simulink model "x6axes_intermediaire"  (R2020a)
settings: Solver=FixedStepAuto  StartTime=0.0  StopTime=t(numel(t))  FixedStep=dt  RelTol=1e-3
model workspace: external: MATLAB File (data not in the file)
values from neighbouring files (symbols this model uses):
  X = [X1(:,1:numel(X1(1,:))-1) X2]    [concat_motion.m]    (also in MGD_6axes.m = [T(1:3,4);Euler]; Trace_6axes.m = [0 0 0; Trace_6axes_trajectoire.m = [0 0 0)
undefined symbols (not defined in the file or in its folder): deg, kg, m, mm, N, rad, s, smiData, Y, Z
libraries: sm_lib x37, nesl_utility x10

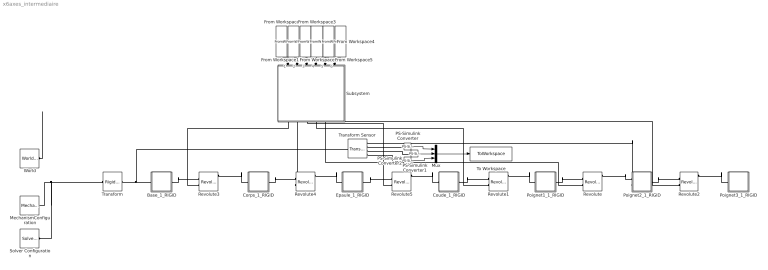
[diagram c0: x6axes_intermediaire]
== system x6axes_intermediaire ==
  Base_1_RIGID : Subsystem
  Corps_1_RIGID : Subsystem
  Coude_1_RIGID : Subsystem
  Epaule_1_RIGID : Subsystem
  From Workspace : FromWorkspace  VariableName=[t' q_targ(1,:)']
  From Workspace1 : FromWorkspace  VariableName=[t' q_targ(2,:)']
  From Workspace2 : FromWorkspace  VariableName=[t' q_targ(3,:)']
  From Workspace3 : FromWorkspace  VariableName=[t' q_targ(4,:)']
  From Workspace4 : FromWorkspace  VariableName=[t' q_targ(5,:)']
  From Workspace5 : FromWorkspace  VariableName=[t' q_targ(6,:)']
  MechanismConfiguration : sm_lib/Utilities/Mechanism Configuration  UniformGravity=Constant  GravityVector=[0 0 -9.80665]  GravityUnits=m/s^2  LinearizationDelta=0.001
  Mux : Mux  Inputs=3
  PS-Simulink Converter : nesl_utility/PS-Simulink Converter  PhysicalDomain=network_engine_domain  SubClassName=ps_output  LeftPortType=input  RightPortType=output  PseudoPeriodic=off  Frequencies=[]  Unit=m  AffineConversion=off
  PS-Simulink Converter1 : nesl_utility/PS-Simulink Converter  PhysicalDomain=network_engine_domain  SubClassName=ps_output  LeftPortType=input  RightPortType=output  PseudoPeriodic=off  Frequencies=[]  Unit=m  AffineConversion=off
  PS-Simulink Converter2 : nesl_utility/PS-Simulink Converter  PhysicalDomain=network_engine_domain  SubClassName=ps_output  LeftPortType=input  RightPortType=output  PseudoPeriodic=off  Frequencies=[]  Unit=m  AffineConversion=off
  Poignet1_1_RIGID : Subsystem
  Poignet2_1_RIGID : Subsystem
  Poignet3_1_RIGID : Subsystem
  Revolute : sm_lib/Joints/Revolute Joint  JointMode=Normal  SenseConstraintForce=off  SenseConstraintForceX=off  SenseConstraintForceY=off  SenseConstraintForceZ=off  SenseConstraintTorque=off  SenseConstraintTorqueX=off  SenseConstraintTorqueY=off  SenseConstraintTorqueZ=off  SenseTotalForce=off  SenseTotalForceX=off  SenseTotalForceY=off  SenseTotalForceZ=off  SenseTotalTorque=off  SenseTotalTorqueX=off  SenseTotalTorqueY=off  SenseTotalTorqueZ=off  CompositeWrenchDir=FollowerOnBase  CompositeWrenchFrame=BaseFrame  EquilibriumPosition=0  EquilibriumPositionUnits=rad  SpringStiffness=0  SpringStiffnessUnits=N*m/rad  DampingCoefficient=0  DampingCoefficientUnits=N*m/(rad/s)  TorqueActuationMode=ComputedTorque  MotionActuationMode=InputMotion  SensePosition=on  SenseVelocity=on  SenseAcceleration=on  SenseTorqueForce=on  SenseLowerLimitTorqueForce=off  SenseUpperLimitTorqueForce=off  LowerLimitSpecify=off  LowerLimitBound=-90  LowerLimitBoundUnits=deg  LowerLimitStiffness=1e4  LowerLimitStiffnessUnits=N*m/deg  LowerLimitDamping=10  LowerLimitDampingUnits=N*m/(deg/s)  LowerLimitTransitionRegionWidth=0.1  LowerLimitTransitionRegionWidthUnits=deg  UpperLimitSpecify=off  UpperLimitBound=90  UpperLimitBoundUnits=deg  UpperLimitStiffness=1e4  UpperLimitStiffnessUnits=N*m/deg  UpperLimitDamping=10  UpperLimitDampingUnits=N*m/(deg/s)  UpperLimitTransitionRegionWidth=0.1  UpperLimitTransitionRegionWidthUnits=deg  PositionTargetSpecify=on  PositionTargetPriority=Low  PositionTargetValue=smiData.RevoluteJoint(1).Rz.Pos  PositionTargetValueUnits=deg  VelocityTargetSpecify=off  VelocityTargetPriority=High  VelocityTargetValue=0  VelocityTargetValueUnits=deg/s
  Revolute1 : sm_lib/Joints/Revolute Joint  JointMode=Normal  SenseConstraintForce=off  SenseConstraintForceX=off  SenseConstraintForceY=off  SenseConstraintForceZ=off  SenseConstraintTorque=off  SenseConstraintTorqueX=off  SenseConstraintTorqueY=off  SenseConstraintTorqueZ=off  SenseTotalForce=off  SenseTotalForceX=off  SenseTotalForceY=off  SenseTotalForceZ=off  SenseTotalTorque=off  SenseTotalTorqueX=off  SenseTotalTorqueY=off  SenseTotalTorqueZ=off  CompositeWrenchDir=FollowerOnBase  CompositeWrenchFrame=BaseFrame  EquilibriumPosition=0  EquilibriumPositionUnits=rad  SpringStiffness=0  SpringStiffnessUnits=N*m/rad  DampingCoefficient=0  DampingCoefficientUnits=N*m/(rad/s)  TorqueActuationMode=ComputedTorque  MotionActuationMode=InputMotion  SensePosition=on  SenseVelocity=on  SenseAcceleration=on  SenseTorqueForce=on  SenseLowerLimitTorqueForce=off  SenseUpperLimitTorqueForce=off  LowerLimitSpecify=off  LowerLimitBound=-90  LowerLimitBoundUnits=deg  LowerLimitStiffness=1e4  LowerLimitStiffnessUnits=N*m/deg  LowerLimitDamping=10  LowerLimitDampingUnits=N*m/(deg/s)  LowerLimitTransitionRegionWidth=0.1  LowerLimitTransitionRegionWidthUnits=deg  UpperLimitSpecify=off  UpperLimitBound=90  UpperLimitBoundUnits=deg  UpperLimitStiffness=1e4  UpperLimitStiffnessUnits=N*m/deg  UpperLimitDamping=10  UpperLimitDampingUnits=N*m/(deg/s)  UpperLimitTransitionRegionWidth=0.1  UpperLimitTransitionRegionWidthUnits=deg  PositionTargetSpecify=on  PositionTargetPriority=Low  PositionTargetValue=smiData.RevoluteJoint(2).Rz.Pos  PositionTargetValueUnits=deg  VelocityTargetSpecify=off  VelocityTargetPriority=High  VelocityTargetValue=0  VelocityTargetValueUnits=deg/s
  Revolute2 : sm_lib/Joints/Revolute Joint  JointMode=Normal  SenseConstraintForce=off  SenseConstraintForceX=off  SenseConstraintForceY=off  SenseConstraintForceZ=off  SenseConstraintTorque=off  SenseConstraintTorqueX=off  SenseConstraintTorqueY=off  SenseConstraintTorqueZ=off  SenseTotalForce=off  SenseTotalForceX=off  SenseTotalForceY=off  SenseTotalForceZ=off  SenseTotalTorque=off  SenseTotalTorqueX=off  SenseTotalTorqueY=off  SenseTotalTorqueZ=off  CompositeWrenchDir=FollowerOnBase  CompositeWrenchFrame=BaseFrame  EquilibriumPosition=0  EquilibriumPositionUnits=rad  SpringStiffness=0  SpringStiffnessUnits=N*m/rad  DampingCoefficient=0  DampingCoefficientUnits=N*m/(rad/s)  TorqueActuationMode=ComputedTorque  MotionActuationMode=InputMotion  SensePosition=on  SenseVelocity=on  SenseAcceleration=on  SenseTorqueForce=on  SenseLowerLimitTorqueForce=off  SenseUpperLimitTorqueForce=off  LowerLimitSpecify=off  LowerLimitBound=-90  LowerLimitBoundUnits=deg  LowerLimitStiffness=1e4  LowerLimitStiffnessUnits=N*m/deg  LowerLimitDamping=10  LowerLimitDampingUnits=N*m/(deg/s)  LowerLimitTransitionRegionWidth=0.1  LowerLimitTransitionRegionWidthUnits=deg  UpperLimitSpecify=off  UpperLimitBound=90  UpperLimitBoundUnits=deg  UpperLimitStiffness=1e4  UpperLimitStiffnessUnits=N*m/deg  UpperLimitDamping=10  UpperLimitDampingUnits=N*m/(deg/s)  UpperLimitTransitionRegionWidth=0.1  UpperLimitTransitionRegionWidthUnits=deg  PositionTargetSpecify=on  PositionTargetPriority=Low  PositionTargetValue=smiData.RevoluteJoint(3).Rz.Pos  PositionTargetValueUnits=deg  VelocityTargetSpecify=off  VelocityTargetPriority=High  VelocityTargetValue=0  VelocityTargetValueUnits=deg/s
  Revolute3 : sm_lib/Joints/Revolute Joint  JointMode=Normal  SenseConstraintForce=off  SenseConstraintForceX=off  SenseConstraintForceY=off  SenseConstraintForceZ=off  SenseConstraintTorque=off  SenseConstraintTorqueX=off  SenseConstraintTorqueY=off  SenseConstraintTorqueZ=off  SenseTotalForce=off  SenseTotalForceX=off  SenseTotalForceY=off  SenseTotalForceZ=off  SenseTotalTorque=off  SenseTotalTorqueX=off  SenseTotalTorqueY=off  SenseTotalTorqueZ=off  CompositeWrenchDir=FollowerOnBase  CompositeWrenchFrame=BaseFrame  EquilibriumPosition=0  EquilibriumPositionUnits=rad  SpringStiffness=0  SpringStiffnessUnits=N*m/rad  DampingCoefficient=0  DampingCoefficientUnits=N*m/(rad/s)  TorqueActuationMode=ComputedTorque  MotionActuationMode=InputMotion  SensePosition=on  SenseVelocity=on  SenseAcceleration=on  SenseTorqueForce=on  SenseLowerLimitTorqueForce=off  SenseUpperLimitTorqueForce=off  LowerLimitSpecify=off  LowerLimitBound=-90  LowerLimitBoundUnits=deg  LowerLimitStiffness=1e4  LowerLimitStiffnessUnits=N*m/deg  LowerLimitDamping=10  LowerLimitDampingUnits=N*m/(deg/s)  LowerLimitTransitionRegionWidth=0.1  LowerLimitTransitionRegionWidthUnits=deg  UpperLimitSpecify=off  UpperLimitBound=90  UpperLimitBoundUnits=deg  UpperLimitStiffness=1e4  UpperLimitStiffnessUnits=N*m/deg  UpperLimitDamping=10  UpperLimitDampingUnits=N*m/(deg/s)  UpperLimitTransitionRegionWidth=0.1  UpperLimitTransitionRegionWidthUnits=deg  PositionTargetSpecify=on  PositionTargetPriority=Low  PositionTargetValue=smiData.RevoluteJoint(4).Rz.Pos  PositionTargetValueUnits=deg  VelocityTargetSpecify=off  VelocityTargetPriority=High  VelocityTargetValue=0  VelocityTargetValueUnits=deg/s
  Revolute4 : sm_lib/Joints/Revolute Joint  JointMode=Normal  SenseConstraintForce=off  SenseConstraintForceX=off  SenseConstraintForceY=off  SenseConstraintForceZ=off  SenseConstraintTorque=off  SenseConstraintTorqueX=off  SenseConstraintTorqueY=off  SenseConstraintTorqueZ=off  SenseTotalForce=off  SenseTotalForceX=off  SenseTotalForceY=off  SenseTotalForceZ=off  SenseTotalTorque=off  SenseTotalTorqueX=off  SenseTotalTorqueY=off  SenseTotalTorqueZ=off  CompositeWrenchDir=FollowerOnBase  CompositeWrenchFrame=BaseFrame  EquilibriumPosition=0  EquilibriumPositionUnits=rad  SpringStiffness=0  SpringStiffnessUnits=N*m/rad  DampingCoefficient=0  DampingCoefficientUnits=N*m/(rad/s)  TorqueActuationMode=ComputedTorque  MotionActuationMode=InputMotion  SensePosition=on  SenseVelocity=on  SenseAcceleration=on  SenseTorqueForce=on  SenseLowerLimitTorqueForce=off  SenseUpperLimitTorqueForce=off  LowerLimitSpecify=off  LowerLimitBound=-90  LowerLimitBoundUnits=deg  LowerLimitStiffness=1e4  LowerLimitStiffnessUnits=N*m/deg  LowerLimitDamping=10  LowerLimitDampingUnits=N*m/(deg/s)  LowerLimitTransitionRegionWidth=0.1  LowerLimitTransitionRegionWidthUnits=deg  UpperLimitSpecify=off  UpperLimitBound=90  UpperLimitBoundUnits=deg  UpperLimitStiffness=1e4  UpperLimitStiffnessUnits=N*m/deg  UpperLimitDamping=10  UpperLimitDampingUnits=N*m/(deg/s)  UpperLimitTransitionRegionWidth=0.1  UpperLimitTransitionRegionWidthUnits=deg  PositionTargetSpecify=on  PositionTargetPriority=Low  PositionTargetValue=smiData.RevoluteJoint(5).Rz.Pos  PositionTargetValueUnits=deg  VelocityTargetSpecify=off  VelocityTargetPriority=High  VelocityTargetValue=0  VelocityTargetValueUnits=deg/s
  Revolute5 : sm_lib/Joints/Revolute Joint  JointMode=Normal  SenseConstraintForce=off  SenseConstraintForceX=off  SenseConstraintForceY=off  SenseConstraintForceZ=off  SenseConstraintTorque=off  SenseConstraintTorqueX=off  SenseConstraintTorqueY=off  SenseConstraintTorqueZ=off  SenseTotalForce=off  SenseTotalForceX=off  SenseTotalForceY=off  SenseTotalForceZ=off  SenseTotalTorque=off  SenseTotalTorqueX=off  SenseTotalTorqueY=off  SenseTotalTorqueZ=off  CompositeWrenchDir=FollowerOnBase  CompositeWrenchFrame=BaseFrame  EquilibriumPosition=0  EquilibriumPositionUnits=rad  SpringStiffness=0  SpringStiffnessUnits=N*m/rad  DampingCoefficient=0  DampingCoefficientUnits=N*m/(rad/s)  TorqueActuationMode=ComputedTorque  MotionActuationMode=InputMotion  SensePosition=on  SenseVelocity=on  SenseAcceleration=on  SenseTorqueForce=on  SenseLowerLimitTorqueForce=off  SenseUpperLimitTorqueForce=off  LowerLimitSpecify=off  LowerLimitBound=-90  LowerLimitBoundUnits=deg  LowerLimitStiffness=1e4  LowerLimitStiffnessUnits=N*m/deg  LowerLimitDamping=10  LowerLimitDampingUnits=N*m/(deg/s)  LowerLimitTransitionRegionWidth=0.1  LowerLimitTransitionRegionWidthUnits=deg  UpperLimitSpecify=off  UpperLimitBound=90  UpperLimitBoundUnits=deg  UpperLimitStiffness=1e4  UpperLimitStiffnessUnits=N*m/deg  UpperLimitDamping=10  UpperLimitDampingUnits=N*m/(deg/s)  UpperLimitTransitionRegionWidth=0.1  UpperLimitTransitionRegionWidthUnits=deg  PositionTargetSpecify=on  PositionTargetPriority=Low  PositionTargetValue=smiData.RevoluteJoint(6).Rz.Pos  PositionTargetValueUnits=deg  VelocityTargetSpecify=off  VelocityTargetPriority=High  VelocityTargetValue=0  VelocityTargetValueUnits=deg/s
  Solver Configuration : nesl_utility/Solver Configuration  PhysicalDomain=network_engine_domain  SubClassName=solver  LeftPortType=input  RightPortType=generic  Tones=[]  Harmonics=[]  SimulateNoise=off  Profile=off  UseLocalSampling=off  EnableSwitchedLinearOptims=on  FrequencyDomain=off  UseCCode=off  RelTol=0.001  AbsTol=1e-06  MinStep=1e-09  ToWorkspace=off  RevertToSquareIcSolve=off  NumHomotopyIterations=100  PhasorMode=off  PhasorModeNumHarmonics=1  DoDC=off  ResidualTolerance=1e-09  UseLocalSolver=off  LocalSolverChoice=NE_BACKWARD_EULER_ADVANCER  LocalSolverSampleTime=0.001  DoFixedCost=off  MaxNonlinIter=3  MaxModeIter=2  LinearAlgebra=auto  EquationFormulation=NE_TIME_EF  DelaysMemoryBudget=1024  AutomaticFiltering=on  FilteringTimeConstant=0.001  PartitionStorageMethod=AS_NEEDED  PartitionMemoryBudget=1024  PartitionMethod=ROBUST
  Subsystem : Subsystem
  To Workspace : ToWorkspace  VariableName=position_poignet  SampleTime=-1
  Transform : sm_lib/Frames and Transforms/Rigid Transform  TranslationMethod=Cartesian  TranslationStandardOffset=0  TranslationLengthUnit=mm  TranslationStandardAxis=+Z  TranslationCartesianOffset=smiData.RigidTransform(10).translation  TranslationROffset=0  TranslationROffsetUnits=m  TranslationZOffset=0  TranslationZOffsetUnits=m  TranslationThetaOffset=0  TranslationThetaOffsetUnits=deg  RotationMethod=ArbitraryAxis  RotationAngleUnits=rad  RotationStandardAxis=+Z  RotationAngle=smiData.RigidTransform(10).angle  RotationArbitraryAxis=smiData.RigidTransform(10).axis  FollAlignAxisA=+X  BaseAlignAxisA=+Y  FollAlignAxisB=+Y  BaseAlignAxisB=+Z  RotationSequenceAxes=FollowerAxes  RotationSequence=XYX  RotationSequenceAngles=[0 0 0]  RotationSequenceAnglesUnits=deg  RotationMatrix=[1 0 0; 0 1 0; 0 0 1]
  Transform Sensor : sm_lib/Frames and Transforms/Transform Sensor  MeasurementFrame=World  SenseAngle=off  SenseAxis=off  SenseAngle1=off  SenseAngle2=off  SenseAngle3=off  SenseQ=off  SenseR=off  SenseOmegaX=off  SenseOmegaY=off  SenseOmegaZ=off  SenseOmega1=off  SenseOmega2=off  SenseOmega3=off  SenseQDot=off  SenseRDot=off  SenseAlphaX=off  SenseAlphaY=off  SenseAlphaZ=off  SenseAlpha1=off  SenseAlpha2=off  SenseAlpha3=off  SenseQDDot=off  SenseRDDot=off  SenseX=on  SenseY=on  SenseZ=on  SenseRad=off  SenseAzim=off  SenseDist=off  SenseInc=off  SenseXDot=off  SenseYDot=off  SenseZDot=off  SenseRadDot=off  SenseAzimDot=off  SenseDistDot=off  SenseIncDot=off  SenseXDDot=off  SenseYDDot=off  SenseZDDot=off  SenseRadDDot=off  SenseAzimDDot=off  SenseDistDDot=off  SenseIncDDot=off
  World : sm_lib/Frames and Transforms/World Frame
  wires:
  PS-Simulink Converter/1 -> Mux/1
  PS-Simulink Converter1/1 -> Mux/2
  PS-Simulink Converter2/1 -> Mux/3
  Mux/1 -> To Workspace/1
  From Workspace2/1 -> Subsystem/3(In3)
  From Workspace1/1 -> Subsystem/2(In2)
  From Workspace3/1 -> Subsystem/4(In4)
  From Workspace5/1 -> Subsystem/6(In6)
  From Workspace/1 -> Subsystem/1(In1)
  From Workspace4/1 -> Subsystem/5(In5)
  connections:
  Transform/LConn1 -- MechanismConfiguration/RConn1 -- Solver Configuration/RConn1 -- World/RConn1
  Poignet1_1_RIGID/RConn1 -- Revolute/LConn1
  Corps_1_RIGID/RConn1 -- Revolute4/LConn1
  Epaule_1_RIGID/LConn1 -- Revolute4/RConn1
  Epaule_1_RIGID/RConn1 -- Revolute5/LConn1
  Coude_1_RIGID/LConn1 -- Revolute5/RConn1
  Poignet2_1_RIGID/LConn1 -- Revolute/RConn1
  Coude_1_RIGID/RConn1 -- Revolute1/LConn1
  Poignet1_1_RIGID/LConn1 -- Revolute1/RConn1
  Poignet2_1_RIGID/RConn1 -- Revolute2/LConn1
  Poignet3_1_RIGID/LConn1 -- Revolute2/RConn1
  Base_1_RIGID/RConn1 -- Revolute3/LConn1
  Corps_1_RIGID/LConn1 -- Revolute3/RConn1
  Base_1_RIGID/LConn1 -- Transform Sensor/LConn1 -- Transform/RConn1
  Poignet2_1_RIGID/LConn2 -- Transform Sensor/RConn1
  PS-Simulink Converter/LConn1 -- Transform Sensor/RConn2
  PS-Simulink Converter2/LConn1 -- Transform Sensor/RConn4
  PS-Simulink Converter1/LConn1 -- Transform Sensor/RConn3
  Subsystem/RConn1 -- Revolute3/LConn2
  Subsystem/RConn2 -- Revolute4/LConn2
  Subsystem/RConn3 -- Revolute5/LConn2
  Subsystem/RConn4 -- Revolute1/LConn2
  Subsystem/RConn5 -- Revolute/LConn2
  Subsystem/RConn6 -- Revolute2/LConn2

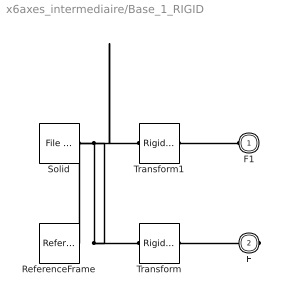
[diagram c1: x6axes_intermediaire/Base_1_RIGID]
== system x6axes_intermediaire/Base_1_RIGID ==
  ReferenceFrame : sm_lib/Frames and Transforms/Reference Frame
  Solid : sm_lib/Body Elements/File Solid  ExtGeomFileName=Base_Défaut_sldprt.STL  UnitType=Custom  ExtGeomFileUnits=mm  StepReaderType=HEX  ExportConvexHullGeometry=off  InertiaType=Custom  Mass=smiData.Solid(3).mass  MassUnits=kg  CenterOfMass=smiData.Solid(3).CoM  CenterOfMassUnits=mm  MomentsOfInertia=smiData.Solid(3).MoI  MomentsOfInertiaUnits=kg*mm^2  ProductsOfInertia=smiData.Solid(3).PoI  ProductsOfInertiaUnits=kg*mm^2  BasedOnType=DensityFromFile  Density=1000  DensityUnits=kg/m^3  DoExposeReferenceFrame=on  SerializedFrames=<Frames/>  GraphicType=FromGeometry  MarkerShape=Sphere  MarkerSize=10  GraphicVisPropType=SimpleVisualProperties  GraphicDiffuseColor=smiData.Solid(3).color  GraphicSpecularColor=[0.5 0.5 0.5 1.0]  GraphicAmbientColor=[0.15 0.15 0.15 1.0]  GraphicEmissiveColor=[0.0 0.0 0.0 1.0]  GraphicShininess=75  GraphicOpacity=smiData.Solid(3).opacity
  Transform : sm_lib/Frames and Transforms/Rigid Transform  TranslationMethod=Cartesian  TranslationStandardOffset=0  TranslationLengthUnit=mm  TranslationStandardAxis=+Z  TranslationCartesianOffset=smiData.RigidTransform(7).translation  TranslationROffset=0  TranslationROffsetUnits=m  TranslationZOffset=0  TranslationZOffsetUnits=m  TranslationThetaOffset=0  TranslationThetaOffsetUnits=deg  RotationMethod=ArbitraryAxis  RotationAngleUnits=rad  RotationStandardAxis=+Z  RotationAngle=smiData.RigidTransform(7).angle  RotationArbitraryAxis=smiData.RigidTransform(7).axis  FollAlignAxisA=+X  BaseAlignAxisA=+Y  FollAlignAxisB=+Y  BaseAlignAxisB=+Z  RotationSequenceAxes=FollowerAxes  RotationSequence=XYX  RotationSequenceAngles=[0 0 0]  RotationSequenceAnglesUnits=deg  RotationMatrix=[1 0 0; 0 1 0; 0 0 1]
  Transform1 : sm_lib/Frames and Transforms/Rigid Transform  TranslationMethod=Cartesian  TranslationStandardOffset=0  TranslationLengthUnit=mm  TranslationStandardAxis=+Z  TranslationCartesianOffset=smiData.RigidTransform(9).translation  TranslationROffset=0  TranslationROffsetUnits=m  TranslationZOffset=0  TranslationZOffsetUnits=m  TranslationThetaOffset=0  TranslationThetaOffsetUnits=deg  RotationMethod=ArbitraryAxis  RotationAngleUnits=rad  RotationStandardAxis=+Z  RotationAngle=smiData.RigidTransform(9).angle  RotationArbitraryAxis=smiData.RigidTransform(9).axis  FollAlignAxisA=+X  BaseAlignAxisA=+Y  FollAlignAxisB=+Y  BaseAlignAxisB=+Z  RotationSequenceAxes=FollowerAxes  RotationSequence=XYX  RotationSequenceAngles=[0 0 0]  RotationSequenceAnglesUnits=deg  RotationMatrix=[1 0 0; 0 1 0; 0 0 1]
  F1 : PMIOPort  Side=Left
  F : PMIOPort  Port=2  Side=Right
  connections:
  Solid/RConn1 -- ReferenceFrame/RConn1 -- Transform/LConn1 -- Transform1/LConn1
  Transform/RConn1 -- F/RConn1
  Transform1/RConn1 -- F1/RConn1

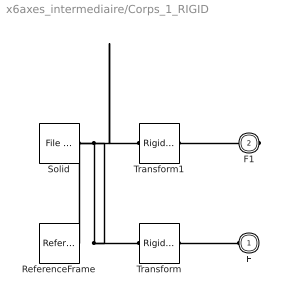
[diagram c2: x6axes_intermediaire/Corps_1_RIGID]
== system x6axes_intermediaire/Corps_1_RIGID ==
  ReferenceFrame : sm_lib/Frames and Transforms/Reference Frame
  Solid : sm_lib/Body Elements/File Solid  ExtGeomFileName=Corps_Défaut_sldprt.STL  UnitType=Custom  ExtGeomFileUnits=mm  StepReaderType=HEX  ExportConvexHullGeometry=off  InertiaType=Custom  Mass=smiData.Solid(2).mass  MassUnits=kg  CenterOfMass=smiData.Solid(2).CoM  CenterOfMassUnits=mm  MomentsOfInertia=smiData.Solid(2).MoI  MomentsOfInertiaUnits=kg*mm^2  ProductsOfInertia=smiData.Solid(2).PoI  ProductsOfInertiaUnits=kg*mm^2  BasedOnType=DensityFromFile  Density=1000  DensityUnits=kg/m^3  DoExposeReferenceFrame=on  SerializedFrames=<Frames/>  GraphicType=FromGeometry  MarkerShape=Sphere  MarkerSize=10  GraphicVisPropType=SimpleVisualProperties  GraphicDiffuseColor=smiData.Solid(2).color  GraphicSpecularColor=[0.5 0.5 0.5 1.0]  GraphicAmbientColor=[0.15 0.15 0.15 1.0]  GraphicEmissiveColor=[0.0 0.0 0.0 1.0]  GraphicShininess=75  GraphicOpacity=smiData.Solid(2).opacity
  Transform : sm_lib/Frames and Transforms/Rigid Transform  TranslationMethod=Cartesian  TranslationStandardOffset=0  TranslationLengthUnit=mm  TranslationStandardAxis=+Z  TranslationCartesianOffset=smiData.RigidTransform(8).translation  TranslationROffset=0  TranslationROffsetUnits=m  TranslationZOffset=0  TranslationZOffsetUnits=m  TranslationThetaOffset=0  TranslationThetaOffsetUnits=deg  RotationMethod=ArbitraryAxis  RotationAngleUnits=rad  RotationStandardAxis=+Z  RotationAngle=smiData.RigidTransform(8).angle  RotationArbitraryAxis=smiData.RigidTransform(8).axis  FollAlignAxisA=+X  BaseAlignAxisA=+Y  FollAlignAxisB=+Y  BaseAlignAxisB=+Z  RotationSequenceAxes=FollowerAxes  RotationSequence=XYX  RotationSequenceAngles=[0 0 0]  RotationSequenceAnglesUnits=deg  RotationMatrix=[1 0 0; 0 1 0; 0 0 1]
  Transform1 : sm_lib/Frames and Transforms/Rigid Transform  TranslationMethod=Cartesian  TranslationStandardOffset=0  TranslationLengthUnit=mm  TranslationStandardAxis=+Z  TranslationCartesianOffset=smiData.RigidTransform(11).translation  TranslationROffset=0  TranslationROffsetUnits=m  TranslationZOffset=0  TranslationZOffsetUnits=m  TranslationThetaOffset=0  TranslationThetaOffsetUnits=deg  RotationMethod=ArbitraryAxis  RotationAngleUnits=rad  RotationStandardAxis=+Z  RotationAngle=smiData.RigidTransform(11).angle  RotationArbitraryAxis=smiData.RigidTransform(11).axis  FollAlignAxisA=+X  BaseAlignAxisA=+Y  FollAlignAxisB=+Y  BaseAlignAxisB=+Z  RotationSequenceAxes=FollowerAxes  RotationSequence=XYX  RotationSequenceAngles=[0 0 0]  RotationSequenceAnglesUnits=deg  RotationMatrix=[1 0 0; 0 1 0; 0 0 1]
  F : PMIOPort  Side=Left
  F1 : PMIOPort  Port=2  Side=Right
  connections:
  Solid/RConn1 -- ReferenceFrame/RConn1 -- Transform/LConn1 -- Transform1/LConn1
  Transform/RConn1 -- F/RConn1
  Transform1/RConn1 -- F1/RConn1

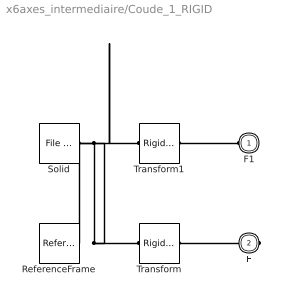
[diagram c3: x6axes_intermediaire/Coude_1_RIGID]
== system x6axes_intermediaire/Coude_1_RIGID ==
  ReferenceFrame : sm_lib/Frames and Transforms/Reference Frame
  Solid : sm_lib/Body Elements/File Solid  ExtGeomFileName=Coude_Défaut_sldprt.STL  UnitType=Custom  ExtGeomFileUnits=mm  StepReaderType=HEX  ExportConvexHullGeometry=off  InertiaType=Custom  Mass=smiData.Solid(5).mass  MassUnits=kg  CenterOfMass=smiData.Solid(5).CoM  CenterOfMassUnits=mm  MomentsOfInertia=smiData.Solid(5).MoI  MomentsOfInertiaUnits=kg*mm^2  ProductsOfInertia=smiData.Solid(5).PoI  ProductsOfInertiaUnits=kg*mm^2  BasedOnType=DensityFromFile  Density=1000  DensityUnits=kg/m^3  DoExposeReferenceFrame=on  SerializedFrames=<Frames/>  GraphicType=FromGeometry  MarkerShape=Sphere  MarkerSize=10  GraphicVisPropType=SimpleVisualProperties  GraphicDiffuseColor=smiData.Solid(5).color  GraphicSpecularColor=[0.5 0.5 0.5 1.0]  GraphicAmbientColor=[0.15 0.15 0.15 1.0]  GraphicEmissiveColor=[0.0 0.0 0.0 1.0]  GraphicShininess=75  GraphicOpacity=smiData.Solid(5).opacity
  Transform : sm_lib/Frames and Transforms/Rigid Transform  TranslationMethod=Cartesian  TranslationStandardOffset=0  TranslationLengthUnit=mm  TranslationStandardAxis=+Z  TranslationCartesianOffset=smiData.RigidTransform(3).translation  TranslationROffset=0  TranslationROffsetUnits=m  TranslationZOffset=0  TranslationZOffsetUnits=m  TranslationThetaOffset=0  TranslationThetaOffsetUnits=deg  RotationMethod=ArbitraryAxis  RotationAngleUnits=rad  RotationStandardAxis=+Z  RotationAngle=smiData.RigidTransform(3).angle  RotationArbitraryAxis=smiData.RigidTransform(3).axis  FollAlignAxisA=+X  BaseAlignAxisA=+Y  FollAlignAxisB=+Y  BaseAlignAxisB=+Z  RotationSequenceAxes=FollowerAxes  RotationSequence=XYX  RotationSequenceAngles=[0 0 0]  RotationSequenceAnglesUnits=deg  RotationMatrix=[1 0 0; 0 1 0; 0 0 1]
  Transform1 : sm_lib/Frames and Transforms/Rigid Transform  TranslationMethod=Cartesian  TranslationStandardOffset=0  TranslationLengthUnit=mm  TranslationStandardAxis=+Z  TranslationCartesianOffset=smiData.RigidTransform(14).translation  TranslationROffset=0  TranslationROffsetUnits=m  TranslationZOffset=0  TranslationZOffsetUnits=m  TranslationThetaOffset=0  TranslationThetaOffsetUnits=deg  RotationMethod=ArbitraryAxis  RotationAngleUnits=rad  RotationStandardAxis=+Z  RotationAngle=smiData.RigidTransform(14).angle  RotationArbitraryAxis=smiData.RigidTransform(14).axis  FollAlignAxisA=+X  BaseAlignAxisA=+Y  FollAlignAxisB=+Y  BaseAlignAxisB=+Z  RotationSequenceAxes=FollowerAxes  RotationSequence=XYX  RotationSequenceAngles=[0 0 0]  RotationSequenceAnglesUnits=deg  RotationMatrix=[1 0 0; 0 1 0; 0 0 1]
  F1 : PMIOPort  Side=Left
  F : PMIOPort  Port=2  Side=Right
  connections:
  Solid/RConn1 -- ReferenceFrame/RConn1 -- Transform/LConn1 -- Transform1/LConn1
  Transform/RConn1 -- F/RConn1
  Transform1/RConn1 -- F1/RConn1

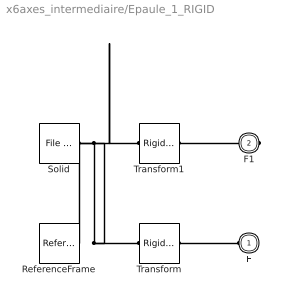
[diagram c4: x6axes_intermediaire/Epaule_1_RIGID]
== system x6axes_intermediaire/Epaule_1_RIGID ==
  ReferenceFrame : sm_lib/Frames and Transforms/Reference Frame
  Solid : sm_lib/Body Elements/File Solid  ExtGeomFileName=Epaule_Défaut_sldprt.STL  UnitType=Custom  ExtGeomFileUnits=mm  StepReaderType=HEX  ExportConvexHullGeometry=off  InertiaType=Custom  Mass=smiData.Solid(7).mass  MassUnits=kg  CenterOfMass=smiData.Solid(7).CoM  CenterOfMassUnits=mm  MomentsOfInertia=smiData.Solid(7).MoI  MomentsOfInertiaUnits=kg*mm^2  ProductsOfInertia=smiData.Solid(7).PoI  ProductsOfInertiaUnits=kg*mm^2  BasedOnType=DensityFromFile  Density=1000  DensityUnits=kg/m^3  DoExposeReferenceFrame=on  SerializedFrames=<Frames/>  GraphicType=FromGeometry  MarkerShape=Sphere  MarkerSize=10  GraphicVisPropType=SimpleVisualProperties  GraphicDiffuseColor=smiData.Solid(7).color  GraphicSpecularColor=[0.5 0.5 0.5 1.0]  GraphicAmbientColor=[0.15 0.15 0.15 1.0]  GraphicEmissiveColor=[0.0 0.0 0.0 1.0]  GraphicShininess=75  GraphicOpacity=smiData.Solid(7).opacity
  Transform : sm_lib/Frames and Transforms/Rigid Transform  TranslationMethod=Cartesian  TranslationStandardOffset=0  TranslationLengthUnit=mm  TranslationStandardAxis=+Z  TranslationCartesianOffset=smiData.RigidTransform(12).translation  TranslationROffset=0  TranslationROffsetUnits=m  TranslationZOffset=0  TranslationZOffsetUnits=m  TranslationThetaOffset=0  TranslationThetaOffsetUnits=deg  RotationMethod=ArbitraryAxis  RotationAngleUnits=rad  RotationStandardAxis=+Z  RotationAngle=smiData.RigidTransform(12).angle  RotationArbitraryAxis=smiData.RigidTransform(12).axis  FollAlignAxisA=+X  BaseAlignAxisA=+Y  FollAlignAxisB=+Y  BaseAlignAxisB=+Z  RotationSequenceAxes=FollowerAxes  RotationSequence=XYX  RotationSequenceAngles=[0 0 0]  RotationSequenceAnglesUnits=deg  RotationMatrix=[1 0 0; 0 1 0; 0 0 1]
  Transform1 : sm_lib/Frames and Transforms/Rigid Transform  TranslationMethod=Cartesian  TranslationStandardOffset=0  TranslationLengthUnit=mm  TranslationStandardAxis=+Z  TranslationCartesianOffset=smiData.RigidTransform(13).translation  TranslationROffset=0  TranslationROffsetUnits=m  TranslationZOffset=0  TranslationZOffsetUnits=m  TranslationThetaOffset=0  TranslationThetaOffsetUnits=deg  RotationMethod=ArbitraryAxis  RotationAngleUnits=rad  RotationStandardAxis=+Z  RotationAngle=smiData.RigidTransform(13).angle  RotationArbitraryAxis=smiData.RigidTransform(13).axis  FollAlignAxisA=+X  BaseAlignAxisA=+Y  FollAlignAxisB=+Y  BaseAlignAxisB=+Z  RotationSequenceAxes=FollowerAxes  RotationSequence=XYX  RotationSequenceAngles=[0 0 0]  RotationSequenceAnglesUnits=deg  RotationMatrix=[1 0 0; 0 1 0; 0 0 1]
  F : PMIOPort  Side=Left
  F1 : PMIOPort  Port=2  Side=Right
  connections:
  Solid/RConn1 -- ReferenceFrame/RConn1 -- Transform/LConn1 -- Transform1/LConn1
  Transform/RConn1 -- F/RConn1
  Transform1/RConn1 -- F1/RConn1

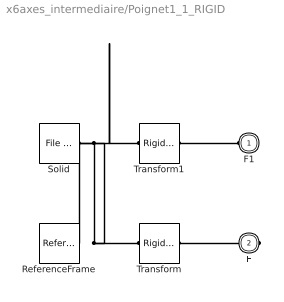
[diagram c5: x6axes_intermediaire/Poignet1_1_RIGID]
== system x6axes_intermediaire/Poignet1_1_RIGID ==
  ReferenceFrame : sm_lib/Frames and Transforms/Reference Frame
  Solid : sm_lib/Body Elements/File Solid  ExtGeomFileName=Poignet1_Défaut_sldprt.STL  UnitType=Custom  ExtGeomFileUnits=mm  StepReaderType=HEX  ExportConvexHullGeometry=off  InertiaType=Custom  Mass=smiData.Solid(6).mass  MassUnits=kg  CenterOfMass=smiData.Solid(6).CoM  CenterOfMassUnits=mm  MomentsOfInertia=smiData.Solid(6).MoI  MomentsOfInertiaUnits=kg*mm^2  ProductsOfInertia=smiData.Solid(6).PoI  ProductsOfInertiaUnits=kg*mm^2  BasedOnType=DensityFromFile  Density=1000  DensityUnits=kg/m^3  DoExposeReferenceFrame=on  SerializedFrames=<Frames/>  GraphicType=FromGeometry  MarkerShape=Sphere  MarkerSize=10  GraphicVisPropType=SimpleVisualProperties  GraphicDiffuseColor=smiData.Solid(6).color  GraphicSpecularColor=[0.5 0.5 0.5 1.0]  GraphicAmbientColor=[0.15 0.15 0.15 1.0]  GraphicEmissiveColor=[0.0 0.0 0.0 1.0]  GraphicShininess=75  GraphicOpacity=smiData.Solid(6).opacity
  Transform : sm_lib/Frames and Transforms/Rigid Transform  TranslationMethod=Cartesian  TranslationStandardOffset=0  TranslationLengthUnit=mm  TranslationStandardAxis=+Z  TranslationCartesianOffset=smiData.RigidTransform(1).translation  TranslationROffset=0  TranslationROffsetUnits=m  TranslationZOffset=0  TranslationZOffsetUnits=m  TranslationThetaOffset=0  TranslationThetaOffsetUnits=deg  RotationMethod=ArbitraryAxis  RotationAngleUnits=rad  RotationStandardAxis=+Z  RotationAngle=smiData.RigidTransform(1).angle  RotationArbitraryAxis=smiData.RigidTransform(1).axis  FollAlignAxisA=+X  BaseAlignAxisA=+Y  FollAlignAxisB=+Y  BaseAlignAxisB=+Z  RotationSequenceAxes=FollowerAxes  RotationSequence=XYX  RotationSequenceAngles=[0 0 0]  RotationSequenceAnglesUnits=deg  RotationMatrix=[1 0 0; 0 1 0; 0 0 1]
  Transform1 : sm_lib/Frames and Transforms/Rigid Transform  TranslationMethod=Cartesian  TranslationStandardOffset=0  TranslationLengthUnit=mm  TranslationStandardAxis=+Z  TranslationCartesianOffset=smiData.RigidTransform(4).translation  TranslationROffset=0  TranslationROffsetUnits=m  TranslationZOffset=0  TranslationZOffsetUnits=m  TranslationThetaOffset=0  TranslationThetaOffsetUnits=deg  RotationMethod=ArbitraryAxis  RotationAngleUnits=rad  RotationStandardAxis=+Z  RotationAngle=smiData.RigidTransform(4).angle  RotationArbitraryAxis=smiData.RigidTransform(4).axis  FollAlignAxisA=+X  BaseAlignAxisA=+Y  FollAlignAxisB=+Y  BaseAlignAxisB=+Z  RotationSequenceAxes=FollowerAxes  RotationSequence=XYX  RotationSequenceAngles=[0 0 0]  RotationSequenceAnglesUnits=deg  RotationMatrix=[1 0 0; 0 1 0; 0 0 1]
  F1 : PMIOPort  Side=Left
  F : PMIOPort  Port=2  Side=Right
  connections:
  Solid/RConn1 -- ReferenceFrame/RConn1 -- Transform/LConn1 -- Transform1/LConn1
  Transform/RConn1 -- F/RConn1
  Transform1/RConn1 -- F1/RConn1

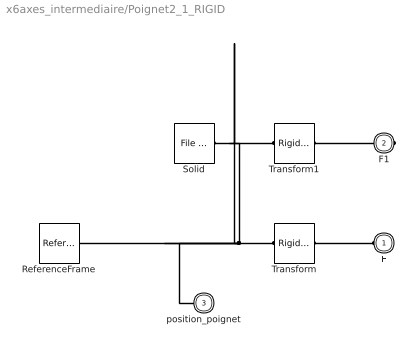
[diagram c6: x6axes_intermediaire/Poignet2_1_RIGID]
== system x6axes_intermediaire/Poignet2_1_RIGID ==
  ReferenceFrame : sm_lib/Frames and Transforms/Reference Frame
  Solid : sm_lib/Body Elements/File Solid  ExtGeomFileName=Poignet2_Défaut_sldprt.STL  UnitType=Custom  ExtGeomFileUnits=mm  StepReaderType=HEX  ExportConvexHullGeometry=off  InertiaType=Custom  Mass=smiData.Solid(1).mass  MassUnits=kg  CenterOfMass=smiData.Solid(1).CoM  CenterOfMassUnits=mm  MomentsOfInertia=smiData.Solid(1).MoI  MomentsOfInertiaUnits=kg*mm^2  ProductsOfInertia=smiData.Solid(1).PoI  ProductsOfInertiaUnits=kg*mm^2  BasedOnType=DensityFromFile  Density=1000  DensityUnits=kg/m^3  DoExposeReferenceFrame=on  SerializedFrames=<Frames/>  GraphicType=FromGeometry  MarkerShape=Sphere  MarkerSize=10  GraphicVisPropType=SimpleVisualProperties  GraphicDiffuseColor=smiData.Solid(1).color  GraphicSpecularColor=[0.5 0.5 0.5 1.0]  GraphicAmbientColor=[0.15 0.15 0.15 1.0]  GraphicEmissiveColor=[0.0 0.0 0.0 1.0]  GraphicShininess=75  GraphicOpacity=smiData.Solid(1).opacity
  Transform : sm_lib/Frames and Transforms/Rigid Transform  TranslationMethod=Cartesian  TranslationStandardOffset=0  TranslationLengthUnit=mm  TranslationStandardAxis=+Z  TranslationCartesianOffset=smiData.RigidTransform(2).translation  TranslationROffset=0  TranslationROffsetUnits=m  TranslationZOffset=0  TranslationZOffsetUnits=m  TranslationThetaOffset=0  TranslationThetaOffsetUnits=deg  RotationMethod=ArbitraryAxis  RotationAngleUnits=rad  RotationStandardAxis=+Z  RotationAngle=smiData.RigidTransform(2).angle  RotationArbitraryAxis=smiData.RigidTransform(2).axis  FollAlignAxisA=+X  BaseAlignAxisA=+Y  FollAlignAxisB=+Y  BaseAlignAxisB=+Z  RotationSequenceAxes=FollowerAxes  RotationSequence=XYX  RotationSequenceAngles=[0 0 0]  RotationSequenceAnglesUnits=deg  RotationMatrix=[1 0 0; 0 1 0; 0 0 1]
  Transform1 : sm_lib/Frames and Transforms/Rigid Transform  TranslationMethod=Cartesian  TranslationStandardOffset=0  TranslationLengthUnit=mm  TranslationStandardAxis=+Z  TranslationCartesianOffset=smiData.RigidTransform(5).translation  TranslationROffset=0  TranslationROffsetUnits=m  TranslationZOffset=0  TranslationZOffsetUnits=m  TranslationThetaOffset=0  TranslationThetaOffsetUnits=deg  RotationMethod=ArbitraryAxis  RotationAngleUnits=rad  RotationStandardAxis=+Z  RotationAngle=smiData.RigidTransform(5).angle  RotationArbitraryAxis=smiData.RigidTransform(5).axis  FollAlignAxisA=+X  BaseAlignAxisA=+Y  FollAlignAxisB=+Y  BaseAlignAxisB=+Z  RotationSequenceAxes=FollowerAxes  RotationSequence=XYX  RotationSequenceAngles=[0 0 0]  RotationSequenceAnglesUnits=deg  RotationMatrix=[1 0 0; 0 1 0; 0 0 1]
  F : PMIOPort  Side=Left
  F1 : PMIOPort  Port=2  Side=Right
  position_poignet : PMIOPort  Port=3  Side=Left
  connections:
  Solid/RConn1 -- position_poignet/RConn1 -- ReferenceFrame/RConn1 -- Transform/LConn1 -- Transform1/LConn1
  Transform/RConn1 -- F/RConn1
  Transform1/RConn1 -- F1/RConn1

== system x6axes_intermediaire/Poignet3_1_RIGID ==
  ReferenceFrame : sm_lib/Frames and Transforms/Reference Frame
  Solid : sm_lib/Body Elements/File Solid  ExtGeomFileName=Poignet3_Défaut_sldprt.STL  UnitType=Custom  ExtGeomFileUnits=mm  StepReaderType=HEX  ExportConvexHullGeometry=off  InertiaType=Custom  Mass=smiData.Solid(4).mass  MassUnits=kg  CenterOfMass=smiData.Solid(4).CoM  CenterOfMassUnits=mm  MomentsOfInertia=smiData.Solid(4).MoI  MomentsOfInertiaUnits=kg*mm^2  ProductsOfInertia=smiData.Solid(4).PoI  ProductsOfInertiaUnits=kg*mm^2  BasedOnType=DensityFromFile  Density=1000  DensityUnits=kg/m^3  DoExposeReferenceFrame=on  SerializedFrames=<Frames/>  GraphicType=FromGeometry  MarkerShape=Sphere  MarkerSize=10  GraphicVisPropType=SimpleVisualProperties  GraphicDiffuseColor=smiData.Solid(4).color  GraphicSpecularColor=[0.5 0.5 0.5 1.0]  GraphicAmbientColor=[0.15 0.15 0.15 1.0]  GraphicEmissiveColor=[0.0 0.0 0.0 1.0]  GraphicShininess=75  GraphicOpacity=smiData.Solid(4).opacity
  Transform : sm_lib/Frames and Transforms/Rigid Transform  TranslationMethod=Cartesian  TranslationStandardOffset=0  TranslationLengthUnit=mm  TranslationStandardAxis=+Z  TranslationCartesianOffset=smiData.RigidTransform(6).translation  TranslationROffset=0  TranslationROffsetUnits=m  TranslationZOffset=0  TranslationZOffsetUnits=m  TranslationThetaOffset=0  TranslationThetaOffsetUnits=deg  RotationMethod=ArbitraryAxis  RotationAngleUnits=rad  RotationStandardAxis=+Z  RotationAngle=smiData.RigidTransform(6).angle  RotationArbitraryAxis=smiData.RigidTransform(6).axis  FollAlignAxisA=+X  BaseAlignAxisA=+Y  FollAlignAxisB=+Y  BaseAlignAxisB=+Z  RotationSequenceAxes=FollowerAxes  RotationSequence=XYX  RotationSequenceAngles=[0 0 0]  RotationSequenceAnglesUnits=deg  RotationMatrix=[1 0 0; 0 1 0; 0 0 1]
  F : PMIOPort  Side=Left
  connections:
  Solid/RConn1 -- ReferenceFrame/RConn1 -- Transform/LConn1
  Transform/RConn1 -- F/RConn1

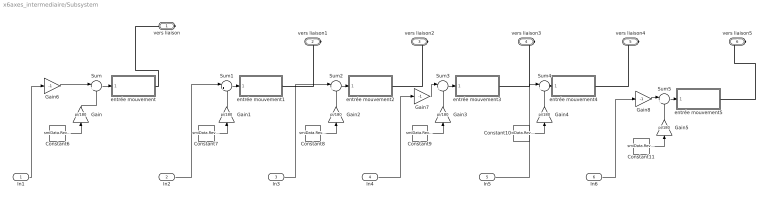
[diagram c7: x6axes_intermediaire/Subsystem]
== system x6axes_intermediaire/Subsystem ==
  In1 : Inport
  In2 : Inport  Port=2
  In3 : Inport  Port=3
  In4 : Inport  Port=4
  In5 : Inport  Port=5
  In6 : Inport  Port=6
  Constant10 : Constant  Value=smiData.RevoluteJoint(1).Rz.Pos
  Constant11 : Constant  Value=smiData.RevoluteJoint(3).Rz.Pos
  Constant6 : Constant  Value=smiData.RevoluteJoint(4).Rz.Pos
  Constant7 : Constant  Value=smiData.RevoluteJoint(5).Rz.Pos
  Constant8 : Constant  Value=smiData.RevoluteJoint(6).Rz.Pos
  Constant9 : Constant  Value=smiData.RevoluteJoint(2).Rz.Pos
  Gain{,1..5} (6 alike) : Gain  Gain=pi/180
  Gain6 : Gain  Gain=-1
  Gain7 : Gain  Gain=-1
  Gain8 : Gain  Gain=-1
  Sum{,1..5} (6 alike) : Sum  Inputs=|++
  entrée mouvement : Subsystem
  entrée mouvement1 : Subsystem
  entrée mouvement2 : Subsystem
  entrée mouvement3 : Subsystem
  entrée mouvement4 : Subsystem
  entrée mouvement5 : Subsystem
  vers liaison : PMIOPort  Side=Right
  vers liaison1 : PMIOPort  Port=2  Side=Right
  vers liaison2 : PMIOPort  Port=3  Side=Right
  vers liaison3 : PMIOPort  Port=4  Side=Right
  vers liaison4 : PMIOPort  Port=5  Side=Right
  vers liaison5 : PMIOPort  Port=6  Side=Right
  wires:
  Constant9/1 -> Gain3/1
  Sum/1 -> entrée mouvement/1(angle)
  Gain2/1 -> Sum2/2
  Sum3/1 -> entrée mouvement3/1(angle)
  Gain1/1 -> Sum1/2
  In6/1 -> Gain8/1
  In1/1 -> Gain6/1
  Sum1/1 -> entrée mouvement1/1(angle)
  Gain4/1 -> Sum4/2
  Gain/1 -> Sum/2
  Sum4/1 -> entrée mouvement4/1(angle)
  Constant7/1 -> Gain1/1
  Sum2/1 -> entrée mouvement2/1(angle)
  Sum5/1 -> entrée mouvement5/1(angle)
  Gain6/1 -> Sum/1
  Gain5/1 -> Sum5/2
  Gain7/1 -> Sum3/1
  Constant8/1 -> Gain2/1
  Gain8/1 -> Sum5/1
  Constant6/1 -> Gain/1
  Gain3/1 -> Sum3/2
  Constant11/1 -> Gain5/1
  Constant10/1 -> Gain4/1
  In5/1 -> Sum4/1
  In4/1 -> Gain7/1
  In2/1 -> Sum1/1
  In3/1 -> Sum2/1
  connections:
  vers liaison3/RConn1 -- entrée mouvement3/RConn1
  vers liaison2/RConn1 -- entrée mouvement2/RConn1
  entrée mouvement/RConn1 -- vers liaison/RConn1
  vers liaison4/RConn1 -- entrée mouvement4/RConn1
  vers liaison1/RConn1 -- entrée mouvement1/RConn1
  vers liaison5/RConn1 -- entrée mouvement5/RConn1

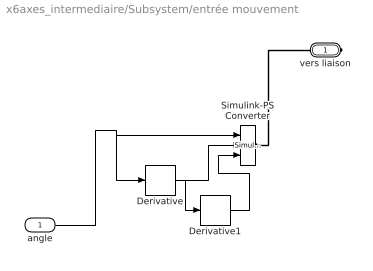
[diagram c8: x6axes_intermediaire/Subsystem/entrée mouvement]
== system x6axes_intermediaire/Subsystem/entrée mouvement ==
  angle : Inport
  Derivative : Derivative
  Derivative1 : Derivative
  Simulink-PS Converter : nesl_utility/Simulink-PS Converter  PhysicalDomain=network_engine_domain  SubClassName=ps_input  LeftPortType=input  RightPortType=output  PseudoPeriodic=off  Frequencies=[]  NoiseDistribution=none  NoiseParameters=[]  Unit=rad  AffineConversion=off  FilteringAndDerivatives=provide  SimscapeFilterOrder=1  InputFilterTimeConstant=0.001  UdotUserProvided=2
  vers liaison : PMIOPort  Side=Right
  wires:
  Derivative/1 -> Simulink-PS Converter/2, Derivative1/1
  Derivative1/1 -> Simulink-PS Converter/3
  angle/1 -> Simulink-PS Converter/1, Derivative/1
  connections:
  Simulink-PS Converter/RConn1 -- vers liaison/RConn1

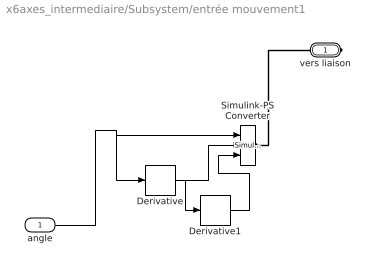
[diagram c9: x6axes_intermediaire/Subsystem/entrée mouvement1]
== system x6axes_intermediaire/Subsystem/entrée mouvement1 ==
  angle : Inport
  Derivative : Derivative
  Derivative1 : Derivative
  Simulink-PS Converter : nesl_utility/Simulink-PS Converter  PhysicalDomain=network_engine_domain  SubClassName=ps_input  LeftPortType=input  RightPortType=output  PseudoPeriodic=off  Frequencies=[]  NoiseDistribution=none  NoiseParameters=[]  Unit=rad  AffineConversion=off  FilteringAndDerivatives=provide  SimscapeFilterOrder=1  InputFilterTimeConstant=0.001  UdotUserProvided=2
  vers liaison : PMIOPort  Side=Right
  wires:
  Derivative/1 -> Simulink-PS Converter/2, Derivative1/1
  Derivative1/1 -> Simulink-PS Converter/3
  angle/1 -> Simulink-PS Converter/1, Derivative/1
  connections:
  Simulink-PS Converter/RConn1 -- vers liaison/RConn1

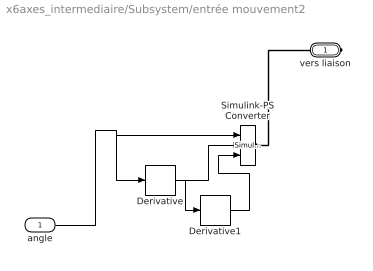
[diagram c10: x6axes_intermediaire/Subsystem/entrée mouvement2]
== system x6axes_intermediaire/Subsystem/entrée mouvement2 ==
  angle : Inport
  Derivative : Derivative
  Derivative1 : Derivative
  Simulink-PS Converter : nesl_utility/Simulink-PS Converter  PhysicalDomain=network_engine_domain  SubClassName=ps_input  LeftPortType=input  RightPortType=output  PseudoPeriodic=off  Frequencies=[]  NoiseDistribution=none  NoiseParameters=[]  Unit=rad  AffineConversion=off  FilteringAndDerivatives=provide  SimscapeFilterOrder=1  InputFilterTimeConstant=0.001  UdotUserProvided=2
  vers liaison : PMIOPort  Side=Right
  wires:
  Derivative/1 -> Simulink-PS Converter/2, Derivative1/1
  Derivative1/1 -> Simulink-PS Converter/3
  angle/1 -> Simulink-PS Converter/1, Derivative/1
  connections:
  Simulink-PS Converter/RConn1 -- vers liaison/RConn1

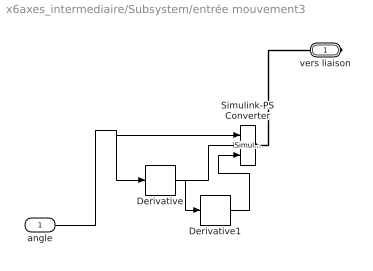
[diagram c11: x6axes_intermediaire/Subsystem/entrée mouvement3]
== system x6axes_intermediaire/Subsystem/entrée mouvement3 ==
  angle : Inport
  Derivative : Derivative
  Derivative1 : Derivative
  Simulink-PS Converter : nesl_utility/Simulink-PS Converter  PhysicalDomain=network_engine_domain  SubClassName=ps_input  LeftPortType=input  RightPortType=output  PseudoPeriodic=off  Frequencies=[]  NoiseDistribution=none  NoiseParameters=[]  Unit=rad  AffineConversion=off  FilteringAndDerivatives=provide  SimscapeFilterOrder=1  InputFilterTimeConstant=0.001  UdotUserProvided=2
  vers liaison : PMIOPort  Side=Right
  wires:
  Derivative/1 -> Simulink-PS Converter/2, Derivative1/1
  Derivative1/1 -> Simulink-PS Converter/3
  angle/1 -> Simulink-PS Converter/1, Derivative/1
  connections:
  Simulink-PS Converter/RConn1 -- vers liaison/RConn1

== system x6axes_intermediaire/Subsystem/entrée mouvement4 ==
  angle : Inport
  Derivative : Derivative
  Derivative1 : Derivative
  Simulink-PS Converter : nesl_utility/Simulink-PS Converter  PhysicalDomain=network_engine_domain  SubClassName=ps_input  LeftPortType=input  RightPortType=output  PseudoPeriodic=off  Frequencies=[]  NoiseDistribution=none  NoiseParameters=[]  Unit=rad  AffineConversion=off  FilteringAndDerivatives=provide  SimscapeFilterOrder=1  InputFilterTimeConstant=0.001  UdotUserProvided=2
  vers liaison : PMIOPort  Side=Right
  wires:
  Derivative/1 -> Simulink-PS Converter/2, Derivative1/1
  Derivative1/1 -> Simulink-PS Converter/3
  angle/1 -> Simulink-PS Converter/1, Derivative/1
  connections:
  Simulink-PS Converter/RConn1 -- vers liaison/RConn1

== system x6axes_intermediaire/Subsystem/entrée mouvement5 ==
  angle : Inport
  Derivative : Derivative
  Derivative1 : Derivative
  Simulink-PS Converter : nesl_utility/Simulink-PS Converter  PhysicalDomain=network_engine_domain  SubClassName=ps_input  LeftPortType=input  RightPortType=output  PseudoPeriodic=off  Frequencies=[]  NoiseDistribution=none  NoiseParameters=[]  Unit=rad  AffineConversion=off  FilteringAndDerivatives=provide  SimscapeFilterOrder=1  InputFilterTimeConstant=0.001  UdotUserProvided=2
  vers liaison : PMIOPort  Side=Right
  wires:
  Derivative/1 -> Simulink-PS Converter/2, Derivative1/1
  Derivative1/1 -> Simulink-PS Converter/3
  angle/1 -> Simulink-PS Converter/1, Derivative/1
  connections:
  Simulink-PS Converter/RConn1 -- vers liaison/RConn1
